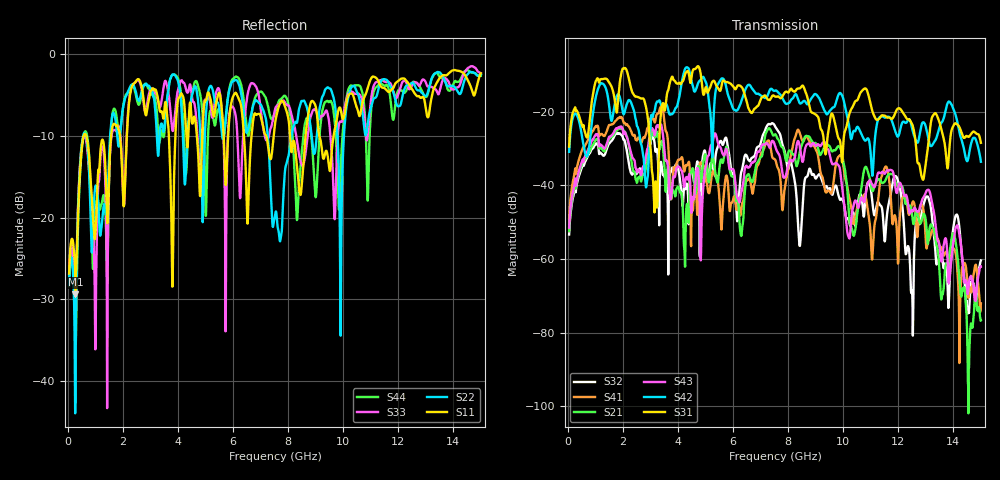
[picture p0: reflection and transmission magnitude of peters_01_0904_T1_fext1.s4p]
# MHZ S RI R 50.00
! FREQ  S11  S12  S13  S14
!  S21  S22  S23  S24
!  S31  S32  S33  S34
!  S41  S42  S43  S44
!  REAL  IMAG  REAL  IMAG  REAL  IMAG  REAL  IMAG
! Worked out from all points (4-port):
!   1496 points, 50 MHz to 15 GHz, reference 50 ohm
!   strongest paths, dB at 50 MHz, 3.79 GHz, 7.53 GHz, 11.27 GHz, 15 GHz:
!     S31: -29.4, -10.4, -15.9, -22.1, -28.4
!     S42: -30.9, -20.6, -14.2, -22.1, -33.6
!     S43: -51.4, -40.6, -29.3, -36.6, -62.0
!     S21: -52.5, -42.0, -26.1, -38.3, -76.7
!     S41: -49.0, -40.9, -33.0, -43.7, -72.1
!     S32: -53.3, -35.2, -24.0, -44.5, -60.4
!   lowest |S11| = -29.4 dB at 280 MHz (marker M1), VSWR 1.07, Z = 53.3 - j1.27 ohm
!   |S11| at or under -10 dB: start of sweep to 581.4 MHz; 674.3 MHz to 1.576 GHz (901.5 MHz wide, 80.1 % of centre); 8.072 GHz to 8.635 GHz (562.5 MHz wide, 6.73 % of centre)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
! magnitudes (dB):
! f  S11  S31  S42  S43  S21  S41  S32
! 50 MHz  -26.8  -29.4  -30.9  -51.4  -52.5  -49.0  -53.3
! 280 MHz  -29.4  -19.3  -20.6  -38.5  -40.6  -36.3  -41.0
! 2.09 GHz  -14.9  -8.1  -19.4  -25.7  -25.6  -23.2  -28.5
! 3.19 GHz  -4.3  -38.9  -18.3  -25.2  -26.8  -22.0  -30.9
! 3.78 GHz  -24.4  -10.5  -20.6  -41.2  -42.6  -42.2  -35.3
! 8.71 GHz  -7.9  -16.3  -18.0  -28.7  -26.6  -27.1  -37.3
! 15 GHz  -2.3  -28.4  -33.6  -62.0  -76.7  -72.1  -60.4
